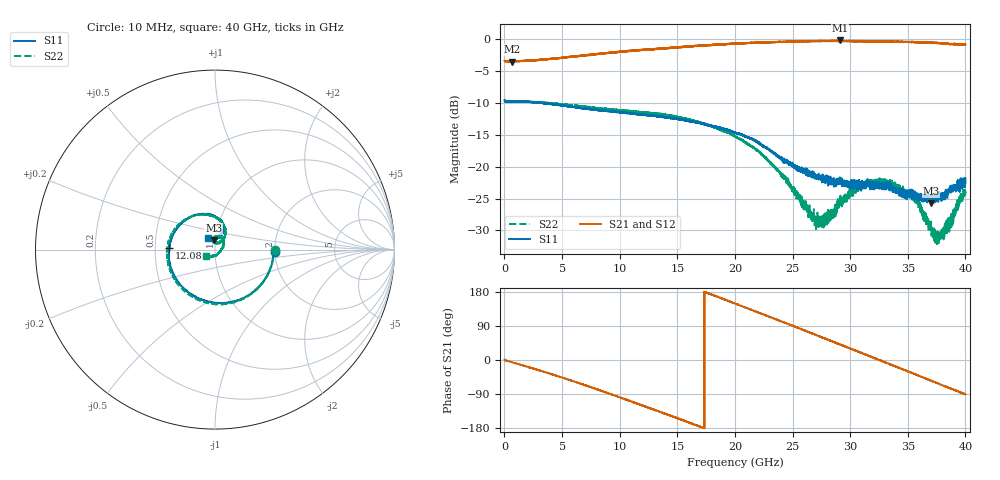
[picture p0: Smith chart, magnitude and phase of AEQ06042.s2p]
! Sonnet Data File
! From: emgraph Version : 16.52
! From Emgraph Data: 3
! Data File Written: 02/28/2018 13:04:54
!< HDATE 02/28/2018 13:03:39
!< MDATE 02/28/2018 13:03:39
# GHZ S MA R 50.00000
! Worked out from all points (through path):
!   6401 points, 10 MHz to 40 GHz, reference 50 ohm
!   highest |S21| = -0.16 dB at 29.12 GHz (marker M1); lowest = -3.5 dB at 622.3 MHz (marker M2)
!   group delay of S21, straight-line fit = 31.7 ps
!   lowest |S11| = -25.7 dB at 37.01 GHz (marker M3), VSWR 1.11, Z = 49.1 + j5.04 ohm
!   |S11| at or under -10 dB: 3.419 GHz to 3.471 GHz (51.71 MHz wide, 1.5 % of centre); 3.472 GHz to 3.52 GHz (47.21 MHz wide, 1.35 % of centre); 3.522 GHz to end of sweep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
!   |S22| runs from -32.5 to -9.5 dB; largest |S21 - S12| = 0.024
!   S11 on the Smith chart (normalised r, x): 10 MHz: 2.00, -0.05; 12.08 GHz: 0.59, +0.01; 40 GHz: 0.92, +0.12
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0.01  0.3347 -2.0  0.6807 1.0  0.6585 0.2  0.3324 -0.2
0.6223469  0.3254 -9.7  0.6704 -5.7  0.6729 -5.6  0.3258 -9.6
3.765311  0.314 -58.4  0.7018 -34.3  0.6998 -34.4  0.3172 -57.8
6.677083  0.2871 -103.2  0.7417 -63.5  0.743 -63.3  0.2977 -101.3
9.48888  0.272 -145.1  0.7902 -92.8  0.7936 -92.9  0.282 -140.6
12.07573  0.2577 178.3  0.8321 -121.1  0.8289 -121.3  0.2663 -175.8
13.34417  0.249 162.0  0.8376 -135.1  0.8425 -135.2  0.2625 167.3
16.91202  0.2206 118.7  0.8964 -175.1  0.8915 -175.0  0.225 123.1
18.49913  0.2044 103.7  0.913 166.5  0.9101 166.8  0.1977 103.4
20.005  0.1846 90.6  0.9275 148.9  0.9284 149.1  0.174 85.2
21.8108  0.1607 75.4  0.9445 127.9  0.9395 127.8  0.1378 66.7
23.62285  0.1255 66.2  0.9562 106.8  0.9567 106.8  0.09577 53.8
25.17871  0.1007 67.1  0.967 88.5  0.9674 88.1  0.06408 54.2
26.67208  0.0877 68.0  0.9708 70.6  0.9727 70.6  0.04269 66.4
27.63434  0.08101 72.3  0.9744 58.9  0.9662 58.9  0.03888 91.2
29.12147  0.07731 74.2  0.9815 40.7  0.9698 41.0  0.0507 104.9
31.27718  0.06918 80.8  0.97 14.8  0.9708 15.1  0.07189 85.5
33.33917  0.07397 82.4  0.9606 -10.0  0.964 -9.8  0.07718 60.7
35.72607  0.05935 87.0  0.9533 -38.7  0.9502 -38.8  0.05197 27.5
37.007  0.05173 97.7  0.9386 -54.0  0.9373 -54.2  0.03323 -11.7
37.83804  0.06039 106.4  0.9308 -64.6  0.9342 -64.8  0.03054 -50.7
40  0.07444 120.6  0.9115 -90.4  0.9119 -90.6  0.06382 -143.1
